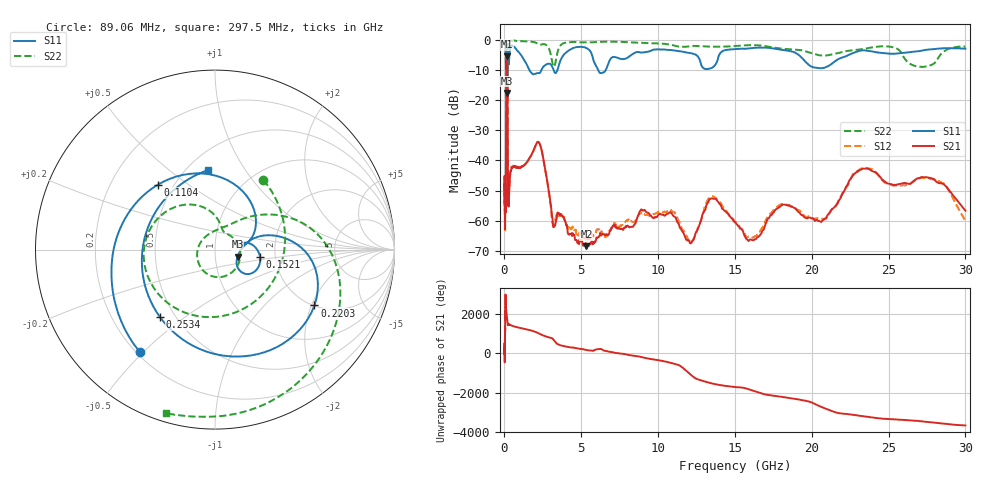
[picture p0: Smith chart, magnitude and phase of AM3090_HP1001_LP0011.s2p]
! Date/Time: Thu, Feb 28, 2019 2:03 PM
! Network Analyzer: Agilent Technologies E8364B Rev: A.07.50.67
! Sweep from 0.010 to 30.000 GHz, 1601 Points, Sweep Type: LOG
! Power Supply: 5.023 V, 0.002 A
# Hz S DB R 50
!freq MagS11 AngS11 MagS21 AngS21 MagS12 AngS12 MagS22 AngS22
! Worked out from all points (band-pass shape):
!   1601 points, 10 MHz to 30 GHz, reference 50 ohm
!   highest |S21| = -5.42 dB at 152.9 MHz (marker M1); lowest = -68.5 dB at 5.338 GHz (marker M2)
!   |S21| within 3 dB of the highest: 123.4 MHz to 191.1 MHz (67.75 MHz wide, 43.1 % of centre)
!   lowest |S11| = -17.6 dB at 185.8 MHz (marker M3), VSWR 1.30, Z = 64.1 - j5.13 ohm
!   |S11| at or under -10 dB: 1.624 GHz to 2.401 GHz (776.3 MHz wide, 38.6 % of centre); 3.201 GHz to 3.449 GHz (247.9 MHz wide, 7.46 % of centre); 6.098 GHz to 6.589 GHz (490.9 MHz wide, 7.74 % of centre)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
!   |S22| runs from -21.0 to -0.2 dB; largest |S21 - S12| = 0.0089
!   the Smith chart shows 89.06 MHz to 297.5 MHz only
!   S11 on the Smith chart (normalised r, x): 89.06 MHz: 0.21, -0.49; 110.4 MHz: 0.41, +0.39; 152.1 MHz: 1.66, -0.14; 220.3 MHz: 2.02, -2.10; 253.4 MHz: 0.41, -0.41; 297.5 MHz: 0.63, +0.70
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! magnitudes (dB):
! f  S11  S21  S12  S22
! 10 MHz  -0.3  -48.0  -46.9  -0.5
! 38.04 MHz  -0.5  -60.6  -61.4  -1.4
! 47.41 MHz  -0.7  -51.4  -47.9  -1.6
! 89.06 MHz  -3.0  -55.9  -52.1  -6.5
! 110.4 MHz  -6.3  -20.1  -20.0  -7.9
! 144.7 MHz  -13.2  -5.5  -5.5  -17.8
! 152.1 MHz  -11.9  -5.4  -5.4  -16.4
! 152.9 MHz  -11.8  -5.4  -5.4  -16.3
! 185.8 MHz  -17.6  -7.3  -7.2  -20.2
! 220.3 MHz  -3.9  -43.3  -44.0  -2.7
! 253.4 MHz  -6.3  -53.5  -53.7  -0.8
! 297.5 MHz  -7.0  -51.6  -50.9  -0.4
! 550.5 MHz  -2.0  -42.1  -42.1  -0.2
! 2.084 GHz  -11.1  -34.4  -34.4  -1.0
! 3.172 GHz  -9.6  -62.1  -60.9  -8.6
! 5.338 GHz  -2.7  -68.5  -66.1  -0.8
! 7.926 GHz  -6.1  -62.1  -60.1  -0.7
! 12.13 GHz  -4.4  -67.5  -66.9  -2.0
! 13.68 GHz  -8.5  -52.7  -52.4  -2.2
! 16.21 GHz  -2.6  -66.5  -65.6  -1.7
! 23.48 GHz  -3.5  -42.7  -42.5  -2.9
! 30 GHz  -2.9  -56.7  -60.1  -2.2
